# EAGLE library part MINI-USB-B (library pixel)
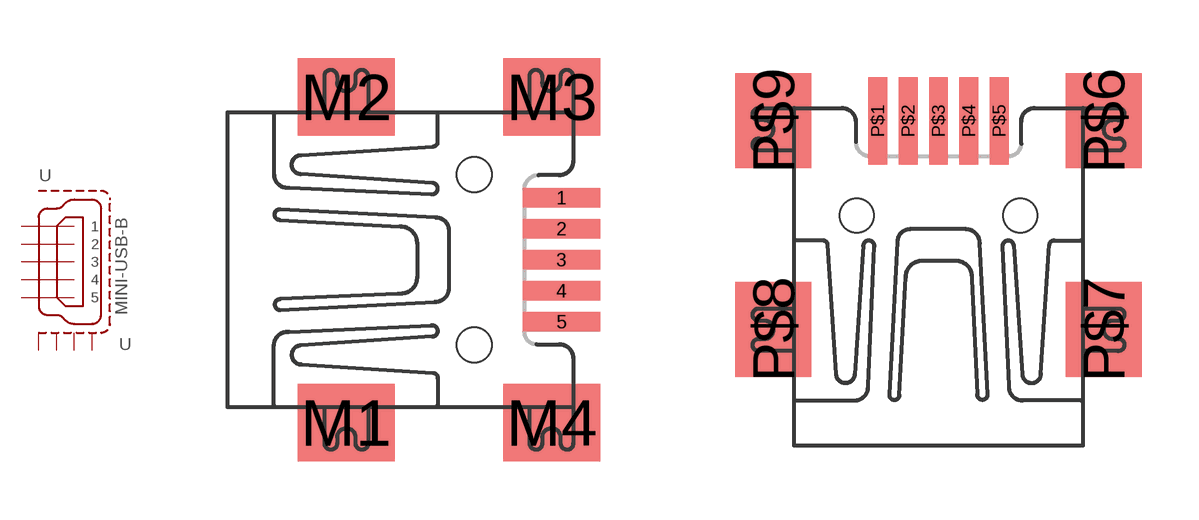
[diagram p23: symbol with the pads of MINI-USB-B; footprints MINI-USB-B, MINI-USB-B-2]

Designator prefix -

## MINI-USB-B  [MINI-USB-B]
1  1  in
2  2  in
3  3  in
4  4  in
5  5  in
M1  S1  pas
M2  S2  pas
M3  S3  pas
M4  S4  pas

## MINI-USB-B2  [MINI-USB-B-2]
P$1  1  in
P$2  2  in
P$3  3  in
P$4  4  in
P$5  5  in
P$6  S1  pas
P$7  S2  pas
P$8  S3  pas
P$9  S4  pas

## Footprint MINI-USB-B (pad centres in mm)
smd 2 x 0.5: 1 2.25,1.6; 2 2.25,0.8; 3 2.25,0; 4 2.25,-0.8; 5 2.25,-1.6
smd 2.5 x 2: M1 -3.3,-4.2; M2 -3.3,4.2; M3 2,4.2; M4 2,-4.2
hole 0.9 at 0,2.2
hole 0.9 at 0,-2.2

## Footprint MINI-USB-B-2 (pad centres in mm)
smd 0.5 x 2.3: P$1 -1.6,2.75; P$2 -0.8,2.75; P$3 0,2.75; P$4 0.8,2.75; P$5 1.6,2.75
smd 2 x 2.5: P$6 4.35,2.75; P$7 4.35,-2.75; P$8 -4.35,-2.75; P$9 -4.35,2.75
hole 0.9 at -2.159,0.254
hole 0.9 at 2.159,0.254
